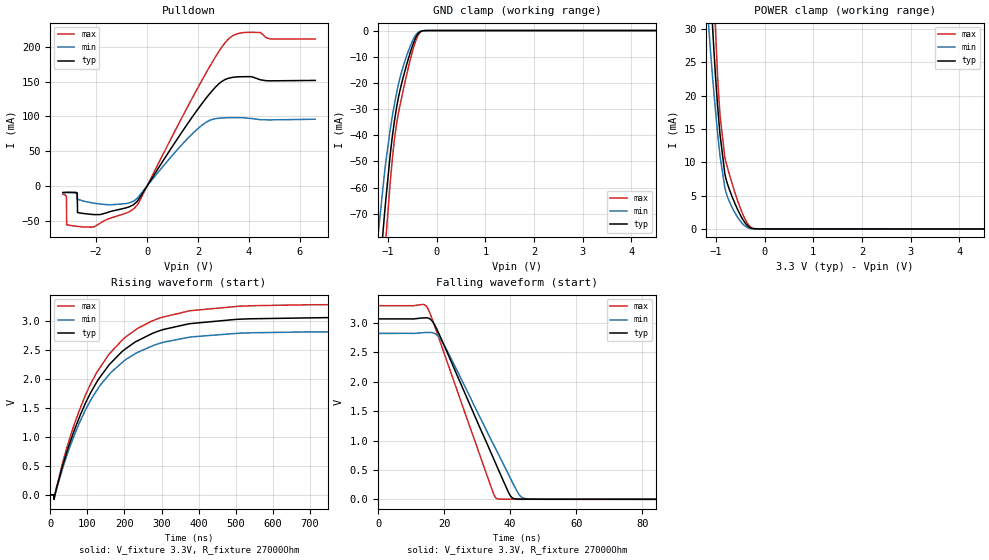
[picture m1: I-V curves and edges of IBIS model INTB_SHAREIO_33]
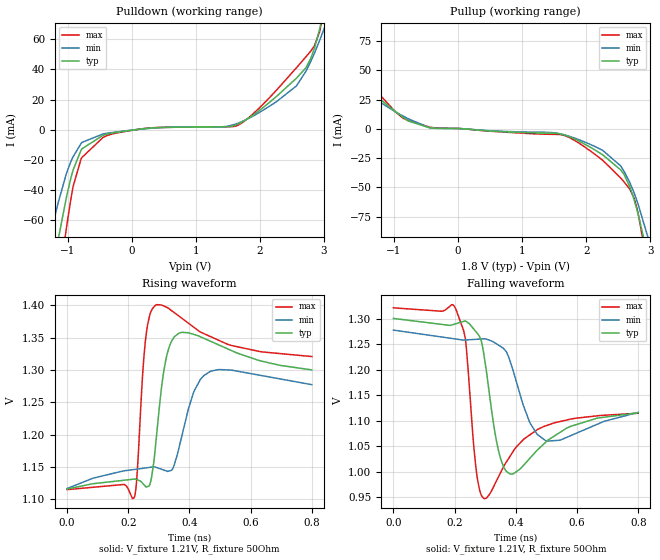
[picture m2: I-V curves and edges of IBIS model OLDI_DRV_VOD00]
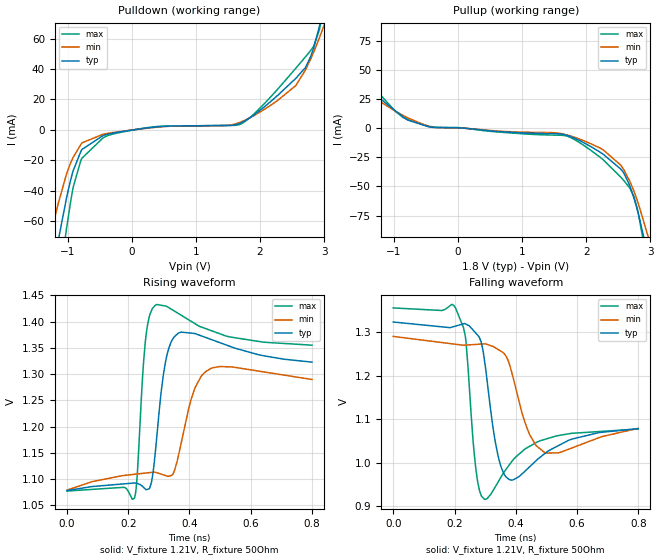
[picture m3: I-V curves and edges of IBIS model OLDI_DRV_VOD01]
|Texas Instruments Incorporated
| Marketing part#   Digital Voltage Range   Package-type   #pins
| DS90UH988-Q1   1.1V-1.8V   QFN   88
[IBIS Ver]   4.1
[File name]   ds90uh988-q1.ibs
[File Rev]   1.1
[Date]   01/30/2026
[Source]
| Texas Instruments Incorporated.
| 12500 TI Blvd
| Dallas, TX -75243
[Notes]   Revision History:
| Rev 1.0: 06/08/2021
| - model generated from design
| - tested RIN0+- as two single ended cells,
| - LVDS_RGB output cell RGB is tested as single ended cells
| Rev 1.1: 01/30/2026
| - model updated to include four OLDI VOD Levels (0,1,2,3)
[Disclaimer]
| This model is designed as an aid for customers of Texas Instruments.
| TI and its licensors and suppliers make no warranties, either expressed
| or implied, with respect to this  model, including the warranties of
| merchantability or fitness for a particular purpose. The model is
| provided solely on an "as is" basis. The entire risk as to its quality
| and performance is with the customer.
[Copyright]
 (C) Copyright 2021 Texas Instruments Incorporated.All rights reserved.
|   Device
[Component]   ds90uh988-q1
[Manufacturer] Texas Instruments
[Package]  |QFN   88
| Package model typ-mean, min, and max
|   typ   min   max
R_pkg   122.9m   104.2m   188.9m
L_pkg   2.03n   1.7n   2.69n
C_pkg   0.405p   0.352p   0.526p
[Pin]  signal_name   model_name   R_pin L_pin C_pin
1   SYNC0   IO_LVCMOS_18  NA   NA   NA
2   SYNC1   IO_LVCMOS_18  NA   NA   NA
3   I2C_SDA1   I2C   NA   NA   NA
4   I2C_SCL1   I2C   NA   NA   NA
5   VDD18_CH1   POWER   NA   NA   NA
6   CH1_TX4P/R0   LVDS_RGB   NA   NA   NA
7   CH1_TX4N/R1   LVDS_RGB   NA   NA   NA
8   CH1_TX3P/R2   LVDS_RGB   NA   NA   NA
9   CH1_TX3N/R3   LVDS_RGB   NA   NA   NA
10   CH1_CLKP/R4   LVDS_RGB   NA   NA   NA
11   CH1_CLKN/R5   LVDS_RGB   NA   NA   NA
12   CH1_TX2P/R6   LVDS_RGB   NA   NA   NA
13   CH1_TX2N/R7   LVDS_RGB   NA   NA   NA
14   CH1_TX1P/G0   LVDS_RGB   NA   NA   NA
15   CH1_TX1N/G1   LVDS_RGB   NA   NA   NA
16   CH1_TX0P/G2   LVDS_RGB   NA   NA   NA
17   CH1_TX0N/G3   LVDS_RGB   NA   NA   NA
18   VDD18_CH1   POWER   NA   NA   NA
19   VDD11_D   POWER   NA   NA   NA
20   VDD18_CHPLL   POWER   NA   NA   NA
21   RBIAS   NC   NA   NA   NA
22   VDD18_CH0   POWER   NA   NA   NA
23   CH0_TX4P/G4   LVDS_RGB   NA   NA   NA
24   CH0_TX4N/G5   LVDS_RGB   NA   NA   NA
25   CH0_TX3P/G6   LVDS_RGB   NA   NA   NA
26   CH0_TX3N/G7   LVDS_RGB   NA   NA   NA
27   CH0_CLKP/B0   LVDS_RGB   NA   NA   NA
28   CH0_CLKP/B1   LVDS_RGB   NA   NA   NA
29   CH0_TX2P/B2   LVDS_RGB   NA   NA   NA
30   CH0_TX2N/B3   LVDS_RGB   NA   NA   NA
31   CH0_TX1P/B4   LVDS_RGB   NA   NA   NA
32   CH0_TX1N/B5   LVDS_RGB   NA   NA   NA
33   CH0_TX0P/B6   LVDS_RGB   NA   NA   NA
34   CH0_TX0N/B7   LVDS_RGB   NA   NA   NA
35   VDD18_CH0   POWER   NA   NA   NA
36   VDD11_TX1PLL   POWER   NA   NA   NA
37   VDD11_TX1   POWER   NA   NA   NA
38   DOUT1-   FPD_TX   NA   NA   NA
39   DOUT1+   FPD_TX   NA   NA   NA
40   VDD18_TXPLL   POWER   NA   NA   NA
41   VDD11_TX0PLL   POWER   NA   NA   NA
42   DOUT0-   FPD_TX   NA   NA   NA
43   DOUT0+   FPD_TX   NA   NA   NA
44   VDD11_TX0   POWER   NA   NA   NA
45   INTB_IN   I_LVCMOS   NA   NA   NA
46   GPIO0   IO_LVCMOS_18  NA   NA   NA
47   GPIO1   IO_LVCMOS_18  NA   NA   NA
48   GPIO2/I2S_DC   IO_LVCMOS_18  NA   NA   NA
49   GPIO3/I2S_DD   IO_LVCMOS_18  NA   NA   NA
50   LOCK0/GPIO4   IO_LVCMOS_18  NA   NA   NA
51   LOCK1/GPIO5/I2S_DB IO_LVCMOS_18  NA   NA   NA
52   LOCK_DUAL/GPIO6/I2S_DA IO_LVCMOS_18  NA   NA   NA
53   GPIO7/I2S_WC   IO_LVCMOS_18  NA   NA   NA
54   GPIO8/I2S_CLK   IO_LVCMOS_18  NA   NA   NA
55   VDD11_D   POWER   NA   NA   NA
56   RES0   NC   NA   NA   NA
57   XO   NC   NA   NA   NA
58   XI   I_XOSC   NA   NA   NA
59   VDD18_D   POWER   NA   NA   NA
60   GPIO9   IO_LVCMOS_18  NA   NA   NA
61   GPIO10/MOSI   IO_LVCMOS_18  NA   NA   NA
62   GPIO11/HS/MISO   IO_LVCMOS_18  NA   NA   NA
63   GPIO12/VS/SPLK   IO_LVCMOS_18  NA   NA   NA
64   GPIO13/DE/SS   IO_LVCMOS_18  NA   NA   NA
65   PCLK/SYNC1   IO_LVCMOS_18  NA   NA   NA
66   ZCLK_IN   IO_LVCMOS_18  NA   NA   NA
67   RES1   NC   NA   NA   NA
68   RES2   NC   NA   NA   NA
69   VDD11_RX0   POWER   NA   NA   NA
70   VDD11_RX0   POWER   NA   NA   NA
71   IDX   NC   NA   NA   NA
72   RIN0+   FPD_RX   NA   NA   NA
73   RIN0-   FPD_RX   NA   NA   NA
74   VDD18_RX0   POWER   NA   NA   NA
75   VDD11_RXPLL   POWER   NA   NA   NA
76   VDD18_RXPLL   POWER   NA   NA   NA
77   VDD11_CML   POWER   NA   NA   NA
78   CMLOUT_P   FPD_TX   NA   NA   NA
79   CMLOUT_N   FPD_TX   NA   NA   NA
80   VDD18_RX1   POWER   NA   NA   NA
81   RIN1+   FPD_RX   NA   NA   NA
82   RIN1-   FPD_RX   NA   NA   NA
83   MODE_SEL0   NC   NA   NA   NA
84   VDD11_RX1   POWER   NA   NA   NA
85   VDD11_RX1   POWER   NA   NA   NA
86   I2C_SDA0   I2C   NA   NA   NA
87   I2C_SCL0   I2C   NA   NA   NA
88   PDB   I_LVCMOS_18   NA   NA   NA
| note: need to comment out diff pairs for RGB output comment out diff pins(6-17,23-34)
| note: FPD-Link receiver pins are tested as single ended inputs, leave commented out
[Diff pin]  inv_pin  vdiff  tdelay_typ  tdelay_min  tdelay_max
6   7   NA   NA   NA   NA
8   9   NA   NA   NA   NA
10   11   NA   NA   NA   NA
12   13   NA   NA   NA   NA
14   15   NA   NA   NA   NA
16   17   NA   NA   NA   NA
23   24   NA   NA   NA   NA
25   26   NA   NA   NA   NA
27   28   NA   NA   NA   NA
29   30   NA   NA   NA   NA
31   32   NA   NA   NA   NA
33   34   NA   NA   NA   NA
38   39   NA   NA   NA   NA
42   43   NA   NA   NA   NA
|72   73   NA   NA   NA   NA
78   79   NA   NA   NA   NA
|81   82   NA   NA   NA   NA
|   Model Selectors
[Model Selector]  I2C
I2C_FAST_18   I2C 400Khz 1.8v
I2C_FASTPLUS_18   I2C 1Mhz   1.8v
I2C_HS_18   I2C 3.4Mhz 1.8v
I2C_FAST_33   I2C 400Khz 3.3v
I2C_FASTPLUS_33   I2C 1Mhz   3.3v
I2C_HS_33   I2C 3.4Mhz 3.3v
[Model Selector]  LVDS_RGB
OLDI_DRV_VOD00   VOD00 OLDI Output
OLDI_DRV_VOD01   VOD01 OLDI Output
OLDI_DRV_VOD10   VOD10 OLDI Output
OLDI_DRV_VOD11   VOD11 OLDI Output
RGB_DRV   RGB 1.8V output
[Model Selector]  FPD_RX
FPD_RX_FPD4   FPD-Link4 Receiver
FPD_RX_FPD3   FPD-Link3 Receiver
[Model Selector]  I_LVCMOS
I_LVCMOS_18   1.8v LVCMOS input
INTB_SHAREIO_33   3.3  LVCMOS input (this is an IO cell, used only for input)
| Models and submodels in the file (18): INTB_SHAREIO_33 (I/O_open_drain), OLDI_DRV_VOD00 (Output), OLDI_DRV_VOD01 (Output), OLDI_DRV_VOD10 (Output), OLDI_DRV_VOD11 (Output), RGB_DRV (Output), FPD_RX_FPD4 (I/O), FPD_RX_FPD3 (I/O), I_XOSC (Input), FPD_TX (Output), I_LVCMOS_18 (Input), I2C_FAST_18 (I/O_open_drain), I2C_FAST_33 (I/O_open_drain), I2C_FASTPLUS_18 (I/O_open_drain), I2C_FASTPLUS_33 (I/O_open_drain), I2C_HS_18 (I/O), I2C_HS_33 (I/O), IO_LVCMOS_18 (I/O)
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| INTB_SHAREIO_33
[Model]   INTB_SHAREIO_33
Model_type   I/O_open_drain
Polarity   Non-Inverting
Enable   Active-High
Vinl = 0.99
Vinh = 2.31
Vmeas = 1.65
Vref = 3.3
Cref = 0pF
Rref = 27000
|   typ   min   max
C_comp   2.908307pF   2.652408pF   3.339183pF
[Voltage Range]   3.3   3   3.6
[Temperature Range]   27   105   -40
[Pullup Reference]   3.3   3   3.6
[Pulldown Reference]   -0   -0   0
[Power Clamp Reference]   3.3   3   3.6
[GND Clamp Reference]   0   0   0
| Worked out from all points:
|   slope of the pulldown table from 0 to 0.495 V, typ, clamps not added: 17.3 ohm
|   GND clamp passes 1 mA (typ) near -0.37 V on its own axis
|   POWER clamp passes 1 mA (typ) near -0.41 V on its own axis
|   falling waveform, V_fixture 3.3V, R_fixture 27000Ohm: 20-80 % time 14.3ns typ, 14.9ns min, 12.3ns max; typ from 3.07 V to 0.002 V
|   rising waveform, V_fixture 3.3V, R_fixture 27000Ohm: 20-80 % time 151ns typ, 150ns min, 150ns max; typ from 0.002 V to 3.07 V
[Pulldown]
|   Voltage   I(typ)   I(min)   I(max)
-3.3V     -9.272mA   -9.512mA   -11.91mA
-3.161V   -9.003mA   -9.27mA    -15.22mA
-3.151V   -8.987mA   -9.256mA   -55.69mA
-2.736V   -10.16mA   -18.57mA   -57.93mA
-2.726V   -38.08mA   -18.76mA   -57.97mA
-2.072V   -40.96mA   -24.59mA   -58.48mA
-676.5mV  -29.45mA   -23.87mA   -36.41mA
-320.1mV  -18.58mA   -14.72mA   -23.24mA
2.095V    115.6mA    85.71mA    148.1mA
3.204V    155mA      98.28mA    211.7mA
4.155V    156.5mA    96.84mA    220.9mA
6.6V      151.8mA    96.02mA    211.3mA
[GND Clamp]
|   Voltage   I(typ)   I(min)   I(max)
-3.3V     -615.5mA   -541.1mA   -700.9mA
-1.211V   -101mA     -79.7mA    -123mA
-1.073V   -70.63mA   -54.78mA   -86.92mA
-1.043V   -64.48mA   -50.08mA   -79.46mA
-933.9mV  -44.27mA   -35.5mA    -54mA
-864.6mV  -34.33mA   -27.91mA   -41.22mA
-815.1mV  -28.59mA   -23.13mA   -34.72mA
-706.2mV  -19.3mA    -14.93mA   -24.48mA
-577.5mV  -10.58mA   -7.646mA   -13.88mA
-458.7mV  -3.987mA   -2.568mA   -5.598mA
-349.8mV  -621.2uA   -387.2uA   -936.6uA
6.6V      0A         0A         0A
[POWER Clamp]
|   Voltage   I(typ)   I(min)   I(max)
-3.3V     554.7mA    458.8mA    658.7mA
-1.142V   42.43mA    29.87mA    59.25mA
-1.063V   29.69mA    22.38mA    40.88mA
-1.013V   23.54mA    18.22mA    30.89mA
-1.003V   22.46mA    17.42mA    29.11mA
-963.6mV  18.48mA    14.37mA    22.91mA
-914.1mV  14.15mA    10.94mA    17.07mA
-815.1mV  8.256mA    6.171mA    10.73mA
-607.2mV  3.804mA    2.414mA    5.429mA
-339.9mV  429uA      182.1uA    727.7uA
-122.1mV  10.85uA    8.314uA    13.88uA
6.6V      0A         0A         0A
[Ramp]
R_load = 27000
|   typ   min   max
dV/dt_r   1.84002/1.51055e-07   1.69213/1.4849e-07   1.9748/1.48829e-07
dV/dt_f   1.84002/1.43251e-08   1.69213/1.49247e-08   1.9748/1.23376e-08
[Falling Waveform]
V_fixture = 3.3V
V_fixture_min = 3V
V_fixture_max = 3.6V
R_fixture = 27000Ohm
C_fixture = 0F
|   Time   V(typ)   V(min)   V(max)
0s        3.069V     2.823V     3.293V
14.75ns   3.087V     2.838V     3.273V
16.69ns   3.007V     2.83V      3.014V
19.69ns   2.657V     2.653V     2.533V
34.77ns   718.8mV    952.5mV    125.9mV
36.74ns   466.8mV    735.7mV    5.5mV
40.56ns   30.35mV    304mV      3.634mV
43.15ns   5.857mV    53.09mV    2.586mV
46.27ns   4.62mV     7.523mV    2.397mV
1.25us    2.119mV    2.437mV    1.85mV
[Rising Waveform]
V_fixture = 3.3V
V_fixture_min = 3V
V_fixture_max = 3.6V
R_fixture = 27000Ohm
C_fixture = 0F
|   Time   V(typ)   V(min)   V(max)
0s        2.119mV    2.437mV    1.85mV
10.16ns   2.211mV    2.544mV    1.922mV
10.31ns   -20.26mV   -3.786mV   -74.77mV
10.52ns   -64.64mV   -75.83mV   -54.04mV
60.78ns   1.048V     966.4mV    1.148V
125.9ns   1.959V     1.814V     2.126V
195ns     2.487V     2.297V     2.686V
273.1ns   2.787V     2.571V     3.005V
509.8ns   3.039V     2.797V     3.264V
1.25us    3.069V     2.823V     3.293V
[Model]   OLDI_DRV_VOD00
Model_type   Output
Polarity   Non-Inverting
Vmeas = 0.55
Vref = 0.55
Cref = 0.02pF
Rref = 50
|   typ   min   max
C_comp   1.47pF   1.46pF   1.53pF
[Voltage Range]   1.8   1.71   1.89
[Temperature Range]   27   105   -40
[Pullup Reference]   1.8   1.71   1.89
[Pulldown Reference]   0   0   0
[Power Clamp Reference]   1.8   1.71   1.89
[GND Clamp Reference]   0   0   0
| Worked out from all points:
|   slope of the pulldown table from 0 to 0.27 V, typ, clamps not added: 203 ohm
|   slope of the pullup table from 0 to 0.27 V, typ, clamps not added: 232 ohm
|   falling waveform, V_fixture 1.21V, R_fixture 50Ohm: 20-80 % time 31.3ps typ, 64.6ps min, 21.8ps max; typ from 1.3 V to 1.12 V
|   rising waveform, V_fixture 1.21V, R_fixture 50Ohm: 20-80 % time 24.3ps typ, 53.7ps min, 14.1ps max; typ from 1.12 V to 1.3 V
[Pulldown]
|   Voltage   I(typ)   I(min)   I(max)
-1.8V     -233mA     -174.7mA   -316.9mA
-1.276V   -103.1mA   -71.27mA   -145.5mA
-1.147V   -72.5mA    -48.12mA   -103.9mA
-1.017V   -44.4mA    -28.68mA   -64.52mA
-914.4mV  -26.61mA   -17.83mA   -37.5mA
-774mV    -12.49mA   -8.255mA   -18.2mA
-244.8mV  -1.736mA   -1.42mA    -2.18mA
1.672V    4.078mA    4.648mA    3.374mA
2.72V     41.15mA    38.92mA    48.48mA
2.936V    67.38mA    59.7mA     65.66mA
3.017V    83.13mA    68.78mA    84.79mA
3.6V      234.9mA    143.1mA    416.1mA
[Pullup]
|   Voltage   I(typ)   I(min)   I(max)
-1.8V     86.89mA    76.05mA    75.83mA
-1.568V   43.58mA    46.96mA    51.44mA
-1.341V   30.88mA    27.14mA    36.35mA
-779.4mV  6.823mA    8.671mA    7.115mA
-369mV    611uA      509.2uA    910.2uA
1.618V    -4.681mA   -4.569mA   -5.077mA
1.975V    -13.05mA   -11.24mA   -15.46mA
2.536V    -35.11mA   -31.7mA    -42.04mA
2.682V    -50.08mA   -46.34mA   -51.92mA
2.812V    -73.76mA   -65.14mA   -73.21mA
3.001V    -118.4mA   -100mA     -130.9mA
3.6V      -271.8mA   -223mA     -334.4mA
[Ramp]
R_load = 50
|   typ   min   max
dV/dt_r   0.110743/2.40942e-11  0.0965742/1.13485e-10   0.123713/1.39939e-11
dV/dt_f   0.110743/3.10429e-11  0.0965742/6.40322e-11   0.123713/2.16623e-11
[Falling Waveform]
V_fixture = 1.21V
V_fixture_min = 1.21V
V_fixture_max = 1.21V
R_fixture = 50Ohm
C_fixture = 0F
|   Time   V(typ)   V(min)   V(max)
0s        1.3V       1.277V     1.321V
203.3ps   1.29V      1.26V      1.32V
235.1ps   1.295V     1.258V     1.261V
268.4ps   1.275V     1.259V     1.015V
295.9ps   1.229V     1.26V      947.8mV
342.9ps   1.043V     1.248V     989.7mV
380.4ps   996.1mV    1.218V     1.03V
444.3ps   1.025V     1.099V     1.072V
497.6ps   1.058V     1.061V     1.09V
800ps     1.116V     1.116V     1.115V
[Rising Waveform]
V_fixture = 1.21V
V_fixture_min = 1.21V
V_fixture_max = 1.21V
R_fixture = 50Ohm
C_fixture = 0F
|   Time   V(typ)   V(min)   V(max)
0s        1.116V     1.116V     1.115V
219.6ps   1.131V     1.146V     1.102V
228.6ps   1.13V      1.146V     1.136V
256ps     1.12V      1.148V     1.344V
288.9ps   1.181V     1.15V      1.4V
322.5ps   1.315V     1.144V     1.398V
365.2ps   1.357V     1.178V     1.384V
416.5ps   1.355V     1.269V     1.366V
466.8ps   1.345V     1.297V     1.352V
800ps     1.3V       1.277V     1.321V
[Model]   OLDI_DRV_VOD01
Model_type   Output
Polarity   Non-Inverting
Vmeas = 0.55
Vref = 0.55
Cref = 0.02pF
Rref = 50
|   typ   min   max
C_comp   1.47pF   1.46pF   1.53pF
[Voltage Range]   1.8   1.71   1.89
[Temperature Range]   27   105   -40
[Pullup Reference]   1.8   1.71   1.89
[Pulldown Reference]   0   0   0
[Power Clamp Reference]   1.8   1.71   1.89
[GND Clamp Reference]   0   0   0
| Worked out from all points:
|   slope of the pulldown table from 0 to 0.27 V, typ, clamps not added: 171 ohm
|   slope of the pullup table from 0 to 0.27 V, typ, clamps not added: 199 ohm
|   falling waveform, V_fixture 1.21V, R_fixture 50Ohm: 20-80 % time 28.8ps typ, 52.8ps min, 19.7ps max; typ from 1.32 V to 1.08 V
|   rising waveform, V_fixture 1.21V, R_fixture 50Ohm: 20-80 % time 25.1ps typ, 49.9ps min, 15.4ps max; typ from 1.08 V to 1.32 V
[Pulldown]
|   Voltage   I(typ)   I(min)   I(max)
-1.8V     -233.6mA   -175.2mA   -317.5mA
-1.276V   -103.6mA   -71.76mA   -146.1mA
-1.147V   -73.01mA   -48.58mA   -104.5mA
-1.017V   -44.87mA   -29.12mA   -65.04mA
-914.4mV  -27.06mA   -18.24mA   -37.99mA
-774mV    -12.88mA   -8.615mA   -18.65mA
-234mV    -1.811mA   -1.491mA   -2.259mA
1.748V    5.463mA    5.934mA    4.869mA
2.709V    40.96mA    39.38mA    48.01mA
2.925V    67.87mA    60.39mA    65.63mA
3.011V    84.84mA    70.13mA    86.59mA
3.6V      238.7mA    145.3mA    423.4mA
[Pullup]
|   Voltage   I(typ)   I(min)   I(max)
-1.8V     86.82mA    75.97mA    75.75mA
-1.568V   43.55mA    46.93mA    51.41mA
-1.346V   31.12mA    27.42mA    36.68mA
-779.4mV  6.823mA    8.67mA     7.115mA
-369mV    611uA      509.1uA    910.2uA
1.667V    -5.728mA   -5.405mA   -6.412mA
1.975V    -12.93mA   -11.13mA   -15.32mA
2.542V    -35.28mA   -31.93mA   -42.2mA
2.682V    -49.89mA   -45.98mA   -51.73mA
2.812V    -73.45mA   -64.7mA    -73.03mA
3.006V    -119.3mA   -100.6mA   -132.4mA
3.6V      -271.3mA   -222.5mA   -334mA
[Ramp]
R_load = 50
|   typ   min   max
dV/dt_r   0.146734/2.50624e-11   0.126423/4.95731e-11   0.166641/1.53376e-11
dV/dt_f   0.146734/2.85269e-11   0.126423/5.22856e-11   0.166641/1.91164e-11
[Falling Waveform]
V_fixture = 1.21V
V_fixture_min = 1.21V
V_fixture_max = 1.21V
R_fixture = 50Ohm
C_fixture = 0F
|   Time   V(typ)   V(min)   V(max)
0s        1.323V     1.29V      1.355V
203.4ps   1.313V     1.272V     1.355V
235ps     1.319V     1.27V      1.292V
268.5ps   1.298V     1.271V     993.6mV
298.1ps   1.234V     1.273V     916.2mV
342.1ps   1.016V     1.26V      955.6mV
380.3ps   961mV      1.224V     996.4mV
442.3ps   988.8mV    1.07V      1.037V
494.6ps   1.021V     1.023V     1.054V
800ps     1.078V     1.079V     1.077V
[Rising Waveform]
V_fixture = 1.21V
V_fixture_min = 1.21V
V_fixture_max = 1.21V
R_fixture = 50Ohm
C_fixture = 0F
|   Time   V(typ)   V(min)   V(max)
0s        1.078V     1.079V     1.077V
219.7ps   1.093V     1.109V     1.063V
228.5ps   1.092V     1.11V      1.101V
255.5ps   1.081V     1.112V     1.36V
288.3ps   1.151V     1.113V     1.431V
322ps     1.324V     1.107V     1.43V
363.8ps   1.378V     1.145V     1.415V
415.2ps   1.378V     1.27V      1.397V
466.6ps   1.367V     1.31V      1.384V
800ps     1.323V     1.29V      1.355V
